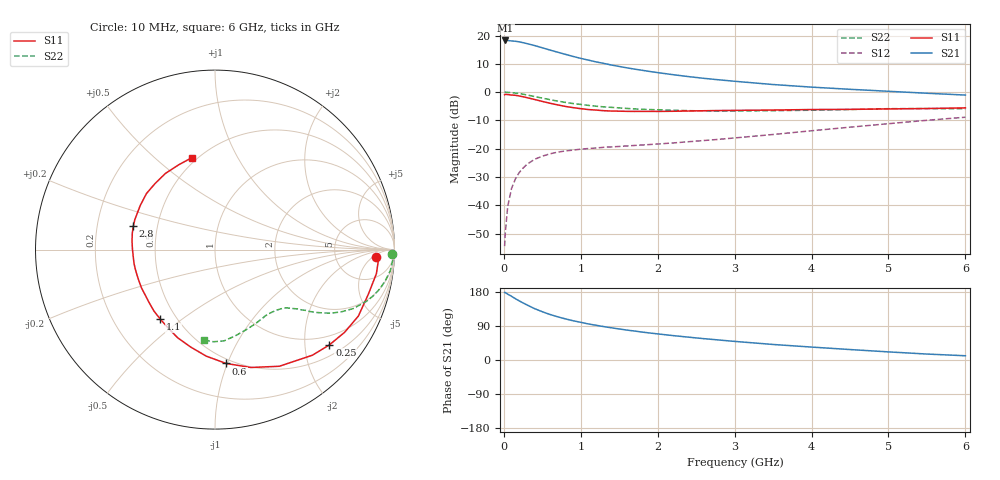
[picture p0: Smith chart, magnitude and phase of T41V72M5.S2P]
! Infineon Technologies  Discrete & RF Semiconductors
! BFR182T
! Si NPN RF Bipolar Junction Transistor in SC75
! VCE = 1.75 V  IC = 2.5 mA
! Common Emitter S-Parameters:  October  1999
# GHz  S  MA  R  50
!  f  S11  S21  S12  S22
! GHz  MAG  ANG  MAG  ANG  MAG  ANG  MAG  ANG
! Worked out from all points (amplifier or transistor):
!   36 points, 10 MHz to 6 GHz, reference 50 ohm
!   highest |S21| = 18.3 dB at 20 MHz (marker M1)
!   |S21| within 3 dB of that: start of sweep to 551.2 MHz
!   unconditionally stable (mu >= 1): 1.803 GHz to 4.32 GHz
!   at 250 MHz: K = 0.17, MSG = 22.2 dB, |S12| = -26.8 dB
!   at 1.4 GHz: K = 0.85, MSG = 14.5 dB, |S12| = -19.3 dB
!   at 6 GHz: K = 0.84, MSG = 3.9 dB, |S12| = -8.8 dB
!   lowest NFmin = 1.10 dB at 450 MHz
!   S11 on the Smith chart (normalised r, x): 10 MHz: 15, -7; 250 MHz: 0.75, -2.57; 600 MHz: 0.46, -0.99; 1.1 GHz: 0.41, -0.42; 2.8 GHz: 0.36, +0.12; 6 GHz: 0.47, +0.67
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0.01  0.898 -2.8  8.148 178.2  0.0019 76.2  0.9881 -1.4
0.02  0.915 -2.0  8.202 177.9  0.0034 93.2  0.9999 -1.5
0.05  0.9091 -8.5  8.186 173.8  0.0095 86.0  0.9915 -3.6
0.1  0.8899 -16.2  8.043 168.1  0.0199 82.2  0.983 -7.0
0.15  0.8804 -24.9  7.939 161.8  0.0292 76.5  0.9646 -10.3
0.2  0.8567 -32.5  7.745 156.0  0.038 73.5  0.9448 -13.3
0.25  0.8296 -39.8  7.493 150.6  0.0456 68.8  0.9194 -16.2
0.3  0.8005 -47.3  7.217 145.3  0.0531 65.8  0.8938 -18.7
0.4  0.7424 -61.1  6.666 135.5  0.0651 59.2  0.8373 -23.1
0.5  0.6865 -73.1  6.087 127.4  0.074 54.7  0.785 -26.2
0.6  0.6374 -84.4  5.551 120.1  0.0814 50.8  0.7374 -28.7
0.8  0.5596 -104.0  4.664 108.5  0.0916 46.0  0.6599 -32.0
0.9  0.5333 -113.0  4.28 103.6  0.0946 44.5  0.6292 -33.2
1.1  0.4929 -128.2  3.683 95.1  0.101 43.2  0.5844 -35.0
1.3  0.4707 -141.4  3.223 88.1  0.1062 42.6  0.5503 -36.7
1.6  0.4582 -158.0  2.688 78.9  0.1122 43.4  0.5158 -39.0
2.2  0.4599 179.8  2.037 64.4  0.1267 48.0  0.4793 -45.1
2.8  0.4737 164.0  1.651 52.7  0.1469 52.5  0.4635 -52.8
3.5  0.4836 149.5  1.365 41.0  0.1787 56.4  0.4711 -62.1
4.5  0.4969 132.3  1.124 27.6  0.2407 57.8  0.4939 -76.9
5.5  0.5139 113.2  0.957 15.7  0.3185 54.8  0.5134 -90.9
6  0.5283 104.0  0.889 11.2  0.3611 51.6  0.5089 -97.2
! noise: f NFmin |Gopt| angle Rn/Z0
0.45  1.1  0.39  29  0.35
0.9  1.2  0.37  59  0.28
1.8  1.8  0.28  128  0.2
